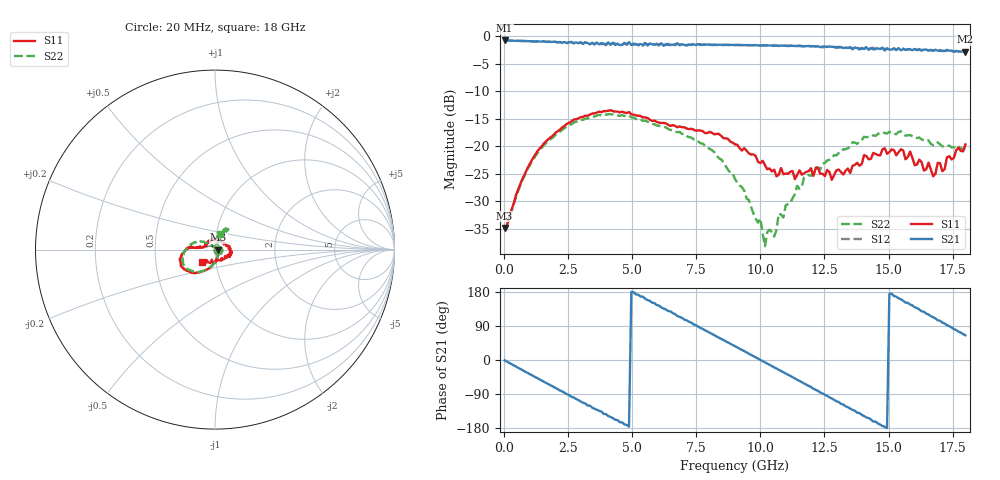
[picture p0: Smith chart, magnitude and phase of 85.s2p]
!Agilent Technologies,N5230A,US43500223,A.07.50.48
!Agilent N5230A: A.07.50.48
!Date: Sunday, January 17, 2016 19:06:15
!Correction: S11(Full 2 Port(1,2))
!S21(Full 2 Port(1,2))
!S12(Full 2 Port(1,2))
!S22(Full 2 Port(1,2))
!S2P File: Measurements: S11, S21, S12, S22:
# Hz S  dB  R 50
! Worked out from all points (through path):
!   201 points, 20 MHz to 18 GHz, reference 50 ohm
!   highest |S21| = -0.78 dB at 20 MHz (marker M1); lowest = -2.8 dB at 18 GHz (marker M2)
!   group delay of S21, straight-line fit = 101 ps
!   lowest |S11| = -34.9 dB at 20 MHz (marker M3), VSWR 1.04, Z = 51.8 - j0.0985 ohm
!   |S11| at or under -10 dB: start of sweep to end of sweep
!   |S22| runs from -38.2 to -14.2 dB; largest |S21 - S12| = 0.037
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2e7  -34.89 -3.0  -0.78 -0.9  -0.78 -0.8  -34.81 -2.1
1.5483e9  -19.52 -105.2  -0.94 -57.2  -0.91 -57.3  -19.86 -105.5
2.3574e9  -16.33 -124.3  -1.08 -86.3  -1.12 -86.2  -16.73 -123.0
3.0766e9  -14.70 -136.3  -1.42 -112.8  -1.34 -112.8  -15.23 -136.7
4.515e9  -13.87 -160.2  -1.63 -164.2  -1.25 -164.6  -14.51 -161.3
4.8746e9  -13.81 -165.4  -1.08 -175.7  -1.23 -174.8  -14.48 -167.1
6.0433e9  -15.73 -179.9  -1.52 143.7  -1.72 142.8  -16.31 175.4
6.7625e9  -16.58 175.5  -1.32 116.1  -1.34 116.6  -17.46 165.6
7.5716e9  -17.14 175.6  -1.45 88.3  -1.47 88.8  -19.18 157.0
9.01e9  -19.68 175.7  -1.61 36.3  -1.62 36.0  -25.97 141.5
9.9989e9  -23.08 170.9  -1.68 0.4  -1.68 0.1  -33.19 118.2
1.01787e10  -23.46 167.2  -1.70 -6.3  -1.69 -6.5  -38.21 105.8
1.03585e10  -24.06 167.3  -1.71 -12.7  -1.68 -13.2  -35.21 98.1
1.05383e10  -24.30 155.5  -1.68 -19.3  -1.76 -19.8  -36.45 88.4
1.07181e10  -25.21 151.8  -1.78 -25.8  -1.77 -26.4  -32.26 82.6
1.08979e10  -25.11 143.0  -1.73 -32.5  -1.66 -32.5  -32.99 74.8
1.20666e10  -25.43 100.8  -1.82 -75.6  -1.84 -75.4  -24.48 67.6
1.3505e10  -24.90 30.5  -2.00 -128.4  -2.10 -127.6  -20.06 66.8
1.50333e10  -21.10 -8.3  -2.45 174.9  -2.40 174.9  -17.38 60.1
1.57525e10  -21.99 -21.8  -2.39 151.0  -2.44 149.3  -18.03 57.6
1.66515e10  -24.28 -73.8  -2.48 115.7  -2.58 114.4  -19.59 63.2
1.8e10  -19.72 -136.0  -2.84 65.1  -2.86 64.0  -20.54 72.3
